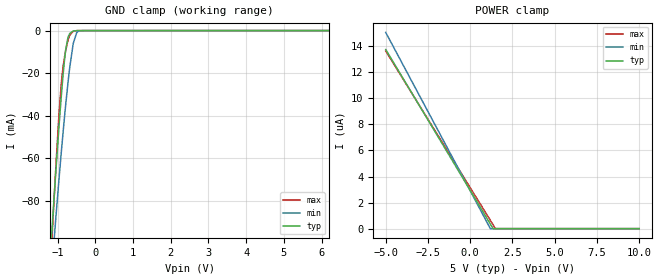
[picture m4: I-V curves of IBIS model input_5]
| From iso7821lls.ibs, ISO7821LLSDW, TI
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|   input_5 Model
[Model]   input_5
Model_type   Input
Vinl = 0.8
Vinh = 2
|   typ   min   max
|   (nom PVT)   (fast PVT)   (slow PVT)
C_comp   3.961e-12   3.930e-12   4.057e-12
| Where nom  PVT is Nominal Process, 5V, 27C
|   Fast PVT is Strong Process,  5.5V, -55C
|   Slow PVT is Weak Process,   4.5V, 150C
[Voltage Range]   5   4.5   5.5
|Junction Temperature
[Temperature Range]   27   150   -55
[Power Clamp Reference]   5   4.5   5.5
[GND Clamp Reference]   0   0   0
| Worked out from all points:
|   GND clamp passes 1 mA (typ) near -0.65 V on its own axis
[GND Clamp]
|   Voltage   I(typ)   I(min)   I(max)
-5V       -1.39A     -1.195A    -1.614A
-1.31V    -138.3mA   -148.4mA   -151.7mA
-1.13V    -87.09mA   -105.7mA   -89.37mA
-1.056V   -67.37mA   -89.07mA   -65.57mA
-960mV    -43.01mA   -68.11mA   -37.23mA
-860mV    -20.78mA   -47.83mA   -17.08mA
-790mV    -8.911mA   -34.77mA   -9.303mA
-730mV    -3.237mA   -24.52mA   -4.588mA
-590mV    -231.2uA   -6.031mA   -312.1uA
-500mV    -40.09uA   -1.038mA   -39.28uA
-356mV    -11uA      -35.76uA   -11.04uA
10V       0A         0A         0A
[POWER Clamp]
|   Voltage   I(typ)   I(min)   I(max)
-5V       13.74uA    15.06uA    13.63uA
1.188V    358.3nA    0A         647.4nA
1.35V     0A         0A         304.6nA
1.49V     0A         0A         0A
10V       0A         0A         0A
